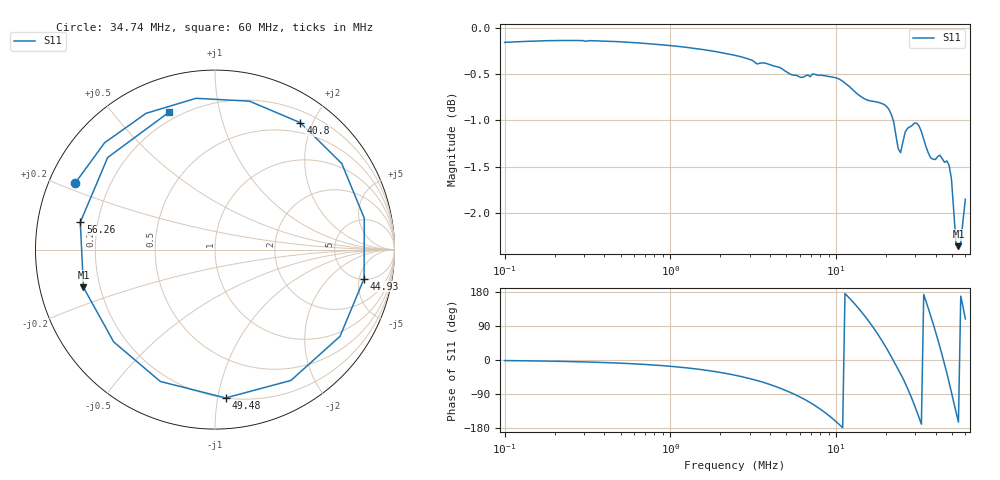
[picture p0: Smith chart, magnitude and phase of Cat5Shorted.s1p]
! ListType=Log
!!Ethernet short VNWA 20s CM
# MHz S DB R 50
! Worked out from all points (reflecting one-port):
!   200 points, 100 kHz to 60 MHz, reference 50 ohm
!   lowest |S11| = -2.4 dB at 54.48 MHz (marker M1), VSWR 7.42, Z = 6.87 - j6.91 ohm
!   phase of S11 starts at -2 deg and turns -970 deg over the sweep
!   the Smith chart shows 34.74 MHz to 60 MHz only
!   S11 on the Smith chart (normalised r, x): 34.74 MHz: 0.08, +0.22; 40.8 MHz: 0.35, +1.83; 44.93 MHz: 5.20, -5.90; 49.48 MHz: 0.20, -1.05; 56.26 MHz: 0.13, +0.10; 60 MHz: 0.16, +0.71
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0.1  -0.16 -1.5
0.2233644  -0.14 -3.7
0.4989166  -0.15 -8.4
1.114402  -0.20 -18.5
2.489178  -0.30 -40.8
5.559937  -0.51 -90.0
8.444173  -0.52 -137.0
10.57502  -0.56 -172.8
12.41892  -0.66 -203.8
14.58434  -0.76 -239.6
16.58551  -0.79 -272.4
18.86128  -0.82 -309.4
21.44931  -0.93 -351.4
24.39246  -1.35 -396.2
27.73945  -1.07 -448.9
29.58142  -1.03 -479.0
31.54569  -1.06 -512.0
34.73935  -1.28 -565.4
38.25634  -1.42 -622.8
40.79665  -1.39 -664.0
43.50565  -1.41 -708.1
44.92688  -1.45 -731.0
47.91013  -1.49 -779.9
49.47524  -1.63 -805.9
51.09148  -1.99 -832.5
54.48407  -2.35 -884.0
56.26394  -2.32 -911.5
60  -1.85 -971.7
